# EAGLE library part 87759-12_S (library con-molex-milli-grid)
HEADER
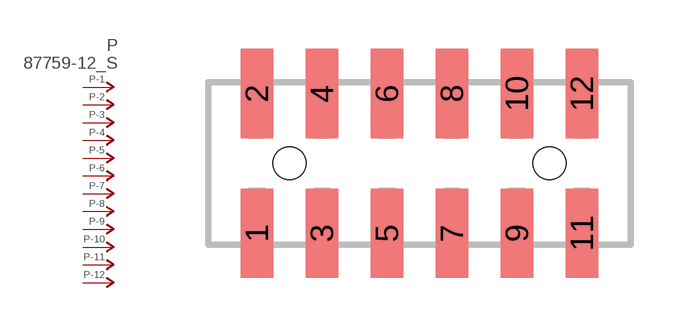
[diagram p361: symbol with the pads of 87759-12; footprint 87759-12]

Designator prefix P; gates -1=P-NV -2=P-N -3=P-N -4=P-N -5=P-N -6=P-N -7=P-N -8=P-N -9=P-N -10=P-N -11=P-N -12=P-N

## 87759-12_S  [87759-12]
1  -1:P  pas
2  -2:P  pas
3  -3:P  pas
4  -4:P  pas
5  -5:P  pas
6  -6:P  pas
7  -7:P  pas
8  -8:P  pas
9  -9:P  pas
10  -10:P  pas
11  -11:P  pas
12  -12:P  pas

## Footprint 87759-12 (pad centres in mm)
HEADER SMD Dual Row, Vertical
smd 1 x 2.75: 1 -5,-2.15; 2 -5,2.15; 3 -3,-2.15; 4 -3,2.15; 5 -1,-2.15; 6 -1,2.15; 7 1,-2.15; 8 1,2.15; 9 3,-2.15; 10 3,2.15; 11 5,-2.15; 12 5,2.15
hole 1 at -4,0
hole 1 at 4,0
